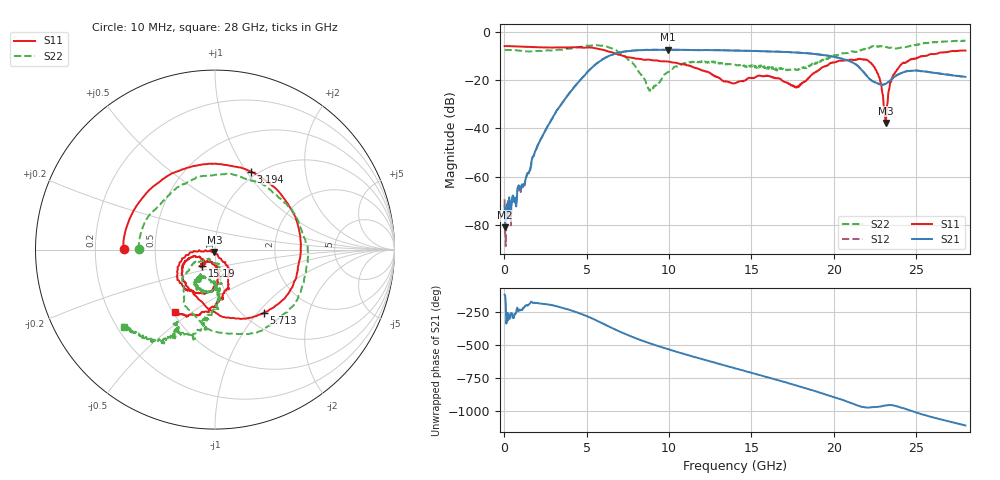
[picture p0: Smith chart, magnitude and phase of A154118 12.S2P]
!  2-Port S-parameters saved by WinCal
! VAR MeasName=S-Parameters (CALIBRATED_DATA) read from VNA (N5230A)
! VAR MeasDate=2015-9-10 14:35:16
! VAR NAME=A154118 12
! VAR FILENAME=A154118 12.S2P
! VAR DATE=2015-9-10 14:35:16
! VAR PHYS_PORTS=1,2
# Hz S DB R 50
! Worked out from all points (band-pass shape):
!   801 points, 10 MHz to 28 GHz, reference 50 ohm
!   highest |S21| = -7.34 dB at 9.911 GHz (marker M1); lowest = -81.0 dB at 44.99 MHz (marker M2)
!   |S21| within 3 dB of the highest: 6.22 GHz to 20.06 GHz (13.84 GHz wide, 105 % of centre)
!   lowest |S11| = -37.7 dB at 23.17 GHz (marker M3), VSWR 1.03, Z = 49.6 - j1.24 ohm
!   |S11| at or under -10 dB: 7.242 GHz to 25.36 GHz (18.11 GHz wide, 111 % of centre); 25.39638 GHz to 25.44811 GHz (51.73 MHz wide, 0.203 % of centre)
!   |S22| runs from -24.5 to -3.5 dB; largest |S21 - S12| = 0.008
!   S11 on the Smith chart (normalised r, x): 10 MHz: 0.32, +0.00; 3.194 GHz: 0.93, +1.05; 5.713 GHz: 1.23, -1.07; 15.19 GHz: 0.86, -0.15; 28 GHz: 0.52, -0.43
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1e7  -5.86 179.6  -72.35 -121.7  -69.44 -33.1  -7.50 179.8
4.49875e7  -5.83 178.5  -81.02 -130.5  -84.44 155.2  -7.46 178.7
1.1296e9  -6.11 141.8  -64.22 137.5  -64.19 134.3  -7.93 146.1
3.193862e9  -6.40 65.3  -32.47 148.5  -32.44 148.6  -7.38 80.2
4.698325e9  -6.43 -4.6  -19.23 90.0  -19.18 89.8  -6.10 12.2
5.712962e9  -7.06 -52.3  -12.55 34.9  -12.49 34.8  -5.57 -42.1
7.182438e9  -9.84 -98.9  -8.25 -51.6  -8.21 -51.7  -9.21 -119.6
8.791862e9  -11.45 -122.3  -7.42 -128.6  -7.37 -129.0  -24.07 -123.1
9.351662e9  -11.92 -130.4  -7.45 -151.7  -7.38 -152.1  -21.68 -76.6
9.911462e9  -12.24 -137.2  -7.34 -173.6  -7.32 -174.0  -16.71 -71.1
1.215066e10  -16.14 -160.8  -7.50 105.6  -7.49 104.9  -12.28 -108.7
1.4005e10  -21.26 -137.7  -7.70 41.0  -7.68 40.6  -13.62 -122.5
1.519458e10  -18.91 -128.0  -7.85 0.5  -7.82 -0.0  -14.17 -114.3
1.774866e10  -22.61 -108.2  -8.53 -89.3  -8.52 -89.9  -15.66 -101.6
1.869332e10  -17.54 -80.9  -9.01 -124.5  -9.02 -124.9  -13.08 -86.2
2.012781e10  -12.39 -99.0  -10.45 179.0  -10.42 178.6  -9.63 -87.6
2.201714e10  -11.67 -143.2  -18.24 104.1  -18.29 103.3  -7.01 -96.2
2.26819e10  -17.22 -174.0  -21.38 110.0  -21.40 109.5  -6.01 -110.1
2.317172e10  -37.73 -106.0  -21.46 121.2  -21.45 121.0  -6.26 -115.6
2.334666e10  -24.22 -56.1  -20.63 123.2  -20.58 123.1  -6.55 -117.4
2.418636e10  -12.95 -70.1  -16.79 101.3  -16.82 100.6  -6.39 -115.0
2.8e10  -7.72 -122.4  -18.62 -30.9  -18.63 -31.5  -3.50 -139.6
